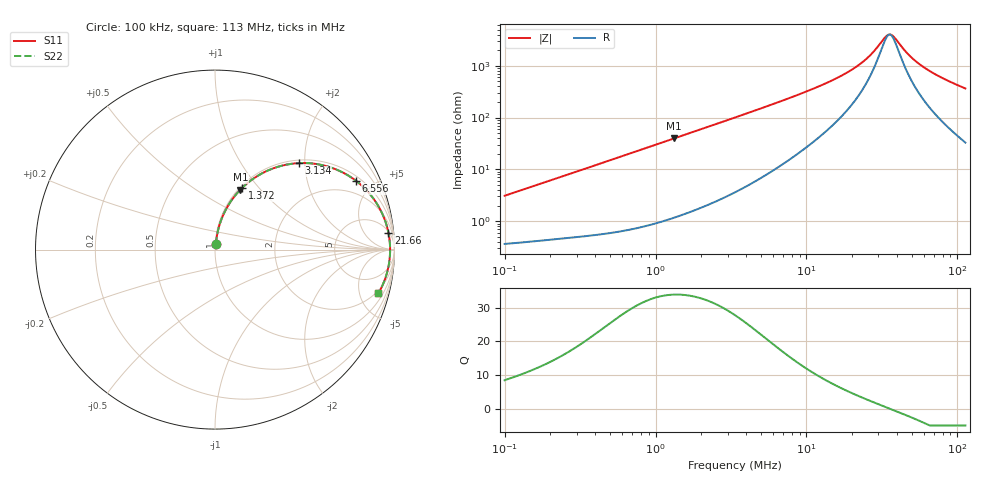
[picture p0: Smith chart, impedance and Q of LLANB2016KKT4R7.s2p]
! LLANB2016KKT4R7  S-PARAMETER MODEL  ( General Type )
! Model Generated by TAIYO YUDEN Corporation (http://www.ty-top.com)
! Version 1.0
! TAIYO YUDEN Control No. 120417NG38SB-FKC
! Copyright(c) 2012 TAIYO YUDEN CO.,LTD. All Rights Reserved.
! Product Description (link to TY-COMPAS)
! https://ds.yuden.co.jp/TYCOMPAS/or/detail?pn=LLANB2016KKT4R7M&u=M
! Products Name : Inductors
! Characteristics :
!  Inductance : 4.7 uH , SRF(min) : -Hz , DC Resistance(max) : 0.38 Ohm
!  Rated Current : Saturation :1000 mA , Temp Rise : 950 mA (40 degC)
!  Case Size : 2.0 x 1.6 / 0.079 x 0.063 [mm/inch] , Thickness : 1 / 0.039 [mm/inch]
!  (Conditions: Temperature = 25 degC , DC Bias Current/Voltage = 0A / 0V)
! External Node Assignments :
!  1  o---GGG---o  2
! GND o---------o GND
! Frequency Range : 0.1MHz  -  113.020708MHz  [ 402 STEP ]
# MHz S RI R 50
! Freq[MHz].  S11 Real  S11 Imag  S21 Real  S21 Imag  S12 Real  S12 Imag  S22 Real  S22 Imag
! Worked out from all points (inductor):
!   401 points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, 100 kHz to 113 MHz, reference 50 ohm
!   read as one part in series: L = 4.86 uH near 103.6 kHz
!   highest Q = 33.9 at 1.324 MHz (marker M1), where L = 4.73 uH
!   self-resonance near 35.6 MHz
!   S11 on the Smith chart (normalised r, x): 100 kHz: 1.01, +0.06; 1.372 MHz: 1.02, +0.82; 3.134 MHz: 1.06, +1.86; 6.556 MHz: 1.22, +3.98; 21.66 MHz: 6, +19; 113 MHz: 1.66, -7.25
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0.1  0.00455 0.0304  0.9955 -0.0304  0.9955 -0.0304  0.00455 0.0304
0.324641  0.0143 0.0957  0.9857 -0.0957  0.9857 -0.0957  0.0143 0.0957
0.590096  0.0359 0.169  0.9641 -0.169  0.9641 -0.169  0.0359 0.169
1.053921  0.0966 0.2808  0.9034 -0.2808  0.9034 -0.2808  0.0966 0.2808
1.32445  0.1416 0.3342  0.8584 -0.3342  0.8584 -0.3342  0.1416 0.3342
1.371833  0.1499 0.3426  0.8501 -0.3426  0.8501 -0.3426  0.1499 0.3426
2.019413  0.2707 0.4293  0.7293 -0.4293  0.7293 -0.4293  0.2707 0.4293
3.133628  0.4659 0.4817  0.5341 -0.4817  0.5341 -0.4817  0.4659 0.4817
3.421463  0.5088 0.4821  0.4912 -0.4821  0.4912 -0.4821  0.5088 0.4821
4.612869  0.6501 0.4559  0.3499 -0.4559  0.3499 -0.4559  0.6501 0.4559
6.55585  0.7864 0.3828  0.2136 -0.3828  0.2136 -0.3828  0.7864 0.3828
10.91398  0.9061 0.2491  0.0939 -0.2491  0.0939 -0.2491  0.9061 0.2491
16.06596  0.9496 0.156  0.0504 -0.156  0.0504 -0.156  0.9496 0.156
21.66037  0.9665 0.0932  0.0335 -0.0932  0.0335 -0.0932  0.9665 0.0932
25.8223  0.972 0.0592  0.028 -0.0592  0.028 -0.0592  0.972 0.0592
33.02595  0.9755 0.0137  0.0245 -0.0137  0.0245 -0.0137  0.9755 0.0137
35.43129  0.9757 0.000863  0.0243 -0.000863  0.0243 -0.000863  0.9757 0.000863
38.01181  0.9756 -0.0119  0.0244 0.0119  0.0244 0.0119  0.9756 -0.0119
47.769  0.9728 -0.0541  0.0272 0.0541  0.0272 0.0541  0.9728 -0.0541
58.98491  0.9665 -0.095  0.0335 0.095  0.0335 0.095  0.9665 -0.095
79.52435  0.9495 -0.1583  0.0505 0.1583  0.0505 0.1583  0.9495 -0.1583
113.0207  0.9109 -0.2432  0.0891 0.2432  0.0891 0.2432  0.9109 -0.2432
